FUNCTION_BLOCK FB_SENT_Decoder
VAR_INPUT
	bEnable					: BOOL;						// enable flag
	nNominalTickTimeUs		: UINT;						// nominal tick time in us
	eFastChannelConfig		: E_SentFastChnConfig;		// layout of the fast-channel data
	eSlowChannelConfig		: E_SentSlowChnConfig;		// layout of the slow-channel data
END_VAR
VAR_OUTPUT
	bNewFrameStart			: BOOL;						// indication flag new frame recieved
	nFrameLenUs				: UINT;						// frame length in µs
	
	bNewFastChnData			: BOOL;						// indication flag new new fast-channel data
	bFastChnDataValid		: BOOL;						// indication flag that the new fast-channel data are valid (CRC)
	nFastChnDataCnt			: UDINT;					// frame-counter of fast-channel data
	
	bNewSlowChnData			: BOOL;						// indication flag new new slow-channel data
	bSlowChnDataValid		: BOOL;						// indication flag that the new slow-channel data are valid (CRC)


	stRawNibbleData			: ST_SentRawNibbleData;		// raw frame data
	stFastChnData			: ST_SentFastChnData;		// last fast-channel data
	stSlowChnData			: ST_SentSlowChnData;		// last slow-channel data
	
	stRxStats				: ST_SentRxStats;			// Recieve statistic
END_VAR
VAR_IN_OUT
	nInputData				: ARRAY[*] OF BOOL;			// input data of the EL1262
END_VAR
VAR
	nMinSyncTimeUs			: UINT;						// nominal sync time - 20%
	nMaxSyncTimeUs			: UINT;						// nominal sync time + 20%
	fActTickTimeUs			: REAL;						// actual tick time (calculated from sync time)
	eFastChnCfgWork			: E_SentFastChnConfig;		// working copy of fast channel layout
	eSlowChnCfgWork			: E_SentSlowChnConfig;		// working conpy of slow channel layout
	bPausePulseWork			: BOOL;						// working copy of pause-pulse config
	nPulsesPerFrame			: UINT;						// number of pulses per send-period (including optional pause pulse)
	                                            		
	bOldValue				: BOOL;						// buffer for detection of falling edge
	bInit					: BOOL := TRUE;				// no falling edge seen yet
	                                            		
	nActSampleCnt			: UINT;						// samples since last falling edge
	nActPulseCnt			: UINT;						// pulses since last sync pulse
	                                            		
	nIdx					: DINT;						// loop-index
	                                            		
	nLowerBoundInput		: DINT;						// lowest index of input-array
	nUpperBoundInput		: DINT;						// highest index of input-array
	nCntInput				: DINT;						// number of elements in input-array
	nstate					: UINT;						// state machine variable
	
	nFastChnCrcCalc			: BYTE;						// calculated crc of fast channel data
	nSlowChnCrcCalc			: BYTE;						// calculated crc of slow channel data

	nNibbleSamples			: ARRAY[1..cMaxPulsesPerFrame] OF UINT;		// array of number of samples for each nibble
	nNibbleTicks			: ARRAY[1..cMaxPulsesPerFrame] OF USINT;	// array of number of ticks for each nibble
	
	nSlowChnBufferB2		: ARRAY[1..cMaxSlowChnLen] OF BOOL;		// Buffer for Status-Bit 2 for slow channel data
	nSlowChnBufferB3		: ARRAY[1..cMaxSlowChnLen] OF BOOL;		// Buffer for Status-Bit 3 for slow channel data
	nShortSlowChnCrcBuff	: ARRAY[1..3] OF USINT;					// Buffer to hold the short slow channel data for CRC calculation
	nEnhSlowChnCrcBuff		: ARRAY[1..4] OF USINT;					// Buffer to hold the enhanced slow channel data for CRC calculation
	
	fbTrigEnable			: Tc2_Standard.R_TRIG;		// edge detection for enable signal
	
	// Testsensor data
	
END_VAR
VAR CONSTANT
	cSyncTicks				: UINT := 56;		// number of ticks in synch pulse
	cMinFactor				: REAL := 0.8;
	cMaxFactor				: REAL := 1.2;
	cMaxPulsesPerFrame		: USINT := 10;
	cMaxSlowChnLen			: USINT := 18;
	
	// todo remove later
	cNibbleOffsetTicks		: UINT := 12;		// number of ticks in nibble für value "0"
	//cMaxNibbleTickLen		: UINT := 35;
	
END_VAR

// check edge on enable signal
fbTrigEnable(CLK:= bEnable);

IF fbTrigEnable.Q THEN
	// calculate min/max sync time
	nMinSyncTimeUs := TO_UINT(TO_REAL(nNominalTickTimeUs * cSyncTicks) * cMinFactor);
	nMaxSyncTimeUs := TO_UINT(TO_REAL(nNominalTickTimeUs * cSyncTicks) * cMaxFactor);
	
	// copy Configdata
	eFastChnCfgWork := eFastChannelConfig;	
	eSlowChnCfgWork := eSlowChannelConfig;
	
	// get number of pulses per frame
	CASE eFastChnCfgWork OF
		E_SentFastChnConfig.eValue_MsgCnt_InvMSB,
		E_SentFastChnConfig.eValue_MsgCnt_Zero,
		E_SentFastChnConfig.eValue_Value:
			nPulsesPerFrame := 9;
		
		E_SentFastChnConfig.eValueCompact:
			nPulsesPerFrame := 6;
		
		E_SentFastChnConfig.eValueExtendet:
			nPulsesPerFrame := 7;
		
	END_CASE
	
	// clear some variables
	fActTickTimeUs := 0.0;
	bInit := TRUE;
	nActPulseCnt := 0;
	Tc2_System.MEMSET(destAddr := ADR(nSlowChnBufferB2), fillByte := 0, n := SIZEOF(nSlowChnBufferB2));
	Tc2_System.MEMSET(destAddr := ADR(nSlowChnBufferB3), fillByte := 0, n := SIZEOF(nSlowChnBufferB3));
END_IF

bNewFrameStart := FALSE;
bNewFastChnData := FALSE;
bFastChnDataValid := FALSE;
bNewSlowChnData := FALSE;
bSlowChnDataValid := FALSE;


IF nInputData <> 0 THEN
	nLowerBoundInput := LOWER_BOUND(nInputData, 1);
	nUpperBoundInput := UPPER_BOUND(nInputData, 1);
	nCntInput := nUpperBoundInput - nLowerBoundInput + 1;
ELSE
	nLowerBoundInput := 0;
	nUpperBoundInput := 0;
	nCntInput := 0;
END_IF;
	
IF nCntInput > 0 THEN
	FOR nIdx := nLowerBoundInput TO nUpperBoundInput DO
		
		IF NOT bInit THEN
			nActSampleCnt := nActSampleCnt + 1;
		END_IF
		
		// check if new falling edge is detected
		IF bOldValue AND NOT nInputData[nIdx] THEN
			bInit := FALSE;
			IF nActSampleCnt > 0 THEN
				IF nMinSyncTimeUs <= nActSampleCnt AND nActSampleCnt <= nMaxSyncTimeUs THEN
					// new sync pulse detected -> clear old data					
					// calculate actual tick time from sync pulse
					fActTickTimeUs := TO_REAL(nActSampleCnt) / TO_REAL(cSyncTicks);
					bNewFrameStart := TRUE;
					nActPulseCnt := 0;
				END_IF
				
				IF fActTickTimeUs > 0.0 THEN
					nActPulseCnt := nActPulseCnt + 1;
					nNibbleSamples[nActPulseCnt] := nActSampleCnt;
					nNibbleTicks[nActPulseCnt] := TO_USINT(TO_REAL(nActSampleCnt) / fActTickTimeUs);
					
					// check if number of pulses (nibbles) is reached -> frame complet received
					IF nActPulseCnt = nPulsesPerFrame THEN
						
						// calculate frame length and update frame statistics
						nFrameLenUs := nNibbleSamples[1] + nNibbleSamples[2] + nNibbleSamples[3] + nNibbleSamples[4] + nNibbleSamples[5] + nNibbleSamples[6] + nNibbleSamples[7] + nNibbleSamples[8] + nNibbleSamples[9] + nNibbleSamples[10];
						stRxStats.nFrmRxCnt := stRxStats.nFrmRxCnt + 1;
						
						// calculate values for the nibbles and the fast channel communication
						M_CalcRawNibbleData();
						M_CalcFastChnData();
						
						bNewFastChnData := TRUE;
						bFastChnDataValid := stFastChnData.nCrc = nFastChnCrcCalc;
						
						IF bNewFastChnData AND bFastChnDataValid THEN
							stRxStats.nFrmRxCntValid := stRxStats.nFrmRxCntValid + 1;
							M_CalcSlowChnData();
						ELSIF  bNewFastChnData AND NOT bFastChnDataValid THEN
							stRxStats.nFrmRxCntInvalid := stRxStats.nFrmRxCntInvalid + 1;
							Tc2_System.MEMSET(destAddr := ADR(nSlowChnBufferB2), fillByte := 0, n := SIZEOF(nSlowChnBufferB2));
							Tc2_System.MEMSET(destAddr := ADR(nSlowChnBufferB3), fillByte := 0, n := SIZEOF(nSlowChnBufferB3));
						END_IF
					END_IF
				END_IF
				nActSampleCnt := 0;
			END_IF
		END_IF
		bOldValue := nInputData[nIdx];
	END_FOR
END_IF

METHOD PRIVATE M_CalcCrc4 : BYTE
VAR_INPUT
END_VAR
VAR_IN_OUT
	aData			: ARRAY[*] OF USINT;
END_VAR
VAR
	nLowBoundData	: DINT;			// lower index
	nUpBoundData	: DINT;			// upper index
	nIdxCntData		: DINT;			// number elements
	
	aCrc4Table 		: ARRAY[0..15] OF BYTE:=[ 0,13,7,10,14,3,9,4,1,12,6,11,15,2,8,5];		// CRC lookup table
	nIdx			: DINT;
	nRetBuff		: BYTE;
END_VAR
// check if input array is not there
IF aData <> 0 THEN
	// get array dimensions 
	nLowBoundData := LOWER_BOUND(aData, 1);
	nUpBoundData := UPPER_BOUND(aData, 1);
	IF nLowBoundData = nUpBoundData THEN
		nIdxCntData := 1;
	ELSE
		nIdxCntData := nUpBoundData - nLowBoundData + 1;	
	END_IF


	nRetBuff:=5;
	
	FOR nIdx := nLowBoundData TO nUpBoundData DO
		nRetBuff := aData[nIdx] XOR aCrc4Table[nRetBuff];
	END_FOR
	
	nRetBuff := 0 XOR aCrc4Table[nRetBuff];

END_IF

 M_CalcCrc4 := nRetBuff;
END_METHOD

METHOD PRIVATE M_CalcCrc4Legacy : BYTE
VAR_INPUT
END_VAR
VAR_IN_OUT
	aData			: ARRAY[*] OF USINT;
END_VAR
VAR
	nLowBoundData	: DINT;			// lower index
	nUpBoundData	: DINT;			// upper index
	nIdxCntData		: DINT;			// number elements
	
	aCrc4Table 		: ARRAY[0..255] OF BYTE:=[	0, 1, 2, 3, 4, 5, 6, 7, 8, 9, 10, 11, 12, 13, 14, 15,
												13, 12, 15, 14, 9, 8, 11, 10, 5, 4, 7, 6, 1, 0, 3, 2,
												7, 6, 5, 4, 3, 2, 1, 0, 15, 14, 13, 12, 11, 10, 9, 8,
												10, 11, 8, 9, 14, 15, 12, 13, 2, 3, 0, 1, 6, 7, 4, 5,
												14, 15, 12, 13, 10, 11, 8, 9, 6, 7, 4, 5, 2, 3, 0, 1,
												3, 2, 1, 0, 7, 6, 5, 4, 11, 10, 9, 8, 15, 14, 13, 12,
												9, 8, 11, 10, 13, 12, 15, 14, 1, 0, 3, 2, 5, 4, 7, 6,
												4, 5, 6, 7, 0, 1, 2, 3, 12, 13, 14, 15, 8, 9, 10, 11,
												1, 0, 3, 2, 5, 4, 7, 6, 9, 8, 11, 10, 13, 12, 15, 14,
												12, 13, 14, 15, 8, 9, 10, 11, 4, 5, 6, 7, 0, 1, 2, 3,
												6, 7, 4, 5, 2, 3, 0, 1, 14, 15, 12, 13, 10, 11, 8, 9,
												11, 10, 9, 8, 15, 14, 13, 12, 3, 2, 1, 0, 7, 6, 5, 4,
												15, 14, 13, 12, 11, 10, 9, 8, 7, 6, 5, 4, 3, 2, 1, 0,
												2, 3, 0, 1, 6, 7, 4, 5, 10, 11, 8, 9, 14, 15, 12, 13,
												8, 9, 10, 11, 12, 13, 14, 15, 0, 1, 2, 3, 4, 5, 6, 7,
												5, 4, 7, 6, 1, 0, 3, 2, 13, 12, 15, 14, 9, 8, 11, 10
												];		// CRC lookup table
	nIdx			: DINT;
	nRetBuff		: BYTE;
	temp			: BYTE;
END_VAR
// check if input array is not there
IF aData <> 0 THEN
	// get array dimensions 
	nLowBoundData := LOWER_BOUND(aData, 1);
	nUpBoundData := UPPER_BOUND(aData, 1);
	IF nLowBoundData = nUpBoundData THEN
		nIdxCntData := 1;
	ELSE
		nIdxCntData := nUpBoundData - nLowBoundData + 1;	
	END_IF


	nRetBuff:=5;
	
	FOR nIdx := nLowBoundData TO nUpBoundData DO
		temp := aData[nIdx] + (nRetBuff * 16);
		nRetBuff := aCrc4Table[temp];
	END_FOR
END_IF

 M_CalcCrc4Legacy := nRetBuff;
END_METHOD

METHOD M_CalcCrc6 : BYTE
VAR_INPUT
END_VAR
VAR_IN_OUT
	aData			: ARRAY[*] OF USINT;
END_VAR
VAR
	nLowBoundData	: DINT;			// lower index
	nUpBoundData	: DINT;			// upper index
	nIdxCntData		: DINT;			// number elements  
	
	aCrc6Table 		: ARRAY[0..63] OF BYTE:=[	0, 25, 50, 43, 61, 36, 15, 22, 35, 58, 17, 8, 30, 7, 44, 53,
												31, 6, 45, 52, 34, 59, 16, 9, 60, 37, 14, 23, 1, 24, 51, 42,
												62, 39, 12, 21, 3, 26, 49, 40, 29, 4, 47, 54, 32, 57, 18, 11,
												33, 56, 19, 10, 28, 5, 46, 55, 2, 27, 48, 41, 63, 38, 13, 20 ];		// CRC lookup table
	nIdx			: DINT;
	nRetBuff		: BYTE;
END_VAR
// check if input array is not there
IF aData <> 0 THEN
	// get array dimensions 
	nLowBoundData := LOWER_BOUND(aData, 1);
	nUpBoundData := UPPER_BOUND(aData, 1);
	IF nLowBoundData = nUpBoundData THEN
		nIdxCntData := 1;
	ELSE
		nIdxCntData := nUpBoundData - nLowBoundData + 1;	
	END_IF

	nRetBuff:=21;
	
	FOR nIdx := nLowBoundData TO nUpBoundData DO
		nRetBuff := aData[nIdx] XOR aCrc6Table[nRetBuff];
	END_FOR
	
	nRetBuff := 0 XOR aCrc6Table[nRetBuff];

END_IF

 M_CalcCrc6 := nRetBuff;
END_METHOD

METHOD PRIVATE M_CalcFastChnData
VAR_INPUT
END_VAR
CASE eFastChnCfgWork OF
	// Status (1 Nibble) + Value_1 (3 Nibble) + Messagecounter (2 Nibble) + invers MSB-Value (1 Nibble) + CRC (1 Nibble)
	E_SentFastChnConfig.eValue_MsgCnt_InvMSB:
		stFastChnData.nStatus := stRawNibbleData.nStatusValue;
		stFastChnData.nValue1 := TO_UINT(stRawNibbleData.nNibbleValue[3])
								+ ROL(TO_UINT(stRawNibbleData.nNibbleValue[2]),4)
								+ ROL(TO_UINT(stRawNibbleData.nNibbleValue[1]),8);
		stFastChnData.nMsgCnt := stRawNibbleData.nNibbleValue[5]
								+ ROL(stRawNibbleData.nNibbleValue[4],4);
		stFastChnData.nInvMsnV1 := stRawNibbleData.nNibbleValue[6];
		stFastChnData.nCrc := stRawNibbleData.nCrcValue;
		
		stFastChnData.nValue2 := 0;
		
	// Status (1 Nibble) + Value_1 (3 Nibble) + Messagecounter (2 Nibble) + Zeros (1 Nibble) + CRC (1 Nibble)
	E_SentFastChnConfig.eValue_MsgCnt_Zero:
		stFastChnData.nStatus := stRawNibbleData.nStatusValue;
		stFastChnData.nValue1 := TO_UINT(stRawNibbleData.nNibbleValue[3])
								+ ROL(TO_UINT(stRawNibbleData.nNibbleValue[2]),4)
								+ ROL(TO_UINT(stRawNibbleData.nNibbleValue[1]),8);
		stFastChnData.nMsgCnt := stRawNibbleData.nNibbleValue[5]
								+ ROL(stRawNibbleData.nNibbleValue[4],4);
		stFastChnData.nCrc := stRawNibbleData.nCrcValue;
		stFastChnData.nInvMsnV1 := 0;
		stFastChnData.nValue2 := 0;
	
	// Status (1 Nibble) + Value_1 (3 Nibble) + Value_2 (3 Nibble) + CRC (1 Nibble)
	E_SentFastChnConfig.eValue_Value:
		stFastChnData.nStatus := stRawNibbleData.nStatusValue;
		stFastChnData.nValue1 := TO_UINT(stRawNibbleData.nNibbleValue[3])
								+ ROL(TO_UINT(stRawNibbleData.nNibbleValue[2]),4)
								+ ROL(TO_UINT(stRawNibbleData.nNibbleValue[1]),8);
		stFastChnData.nValue2 := TO_UINT(stRawNibbleData.nNibbleValue[6])
								+ ROL(TO_UINT(stRawNibbleData.nNibbleValue[5]),4)
								+ ROL(TO_UINT(stRawNibbleData.nNibbleValue[4]),8);
		stFastChnData.nCrc := stRawNibbleData.nCrcValue;
		
		stFastChnData.nMsgCnt := 0;
		stFastChnData.nInvMsnV1 := 0;
	
	// Status (1 Nibble) + Value_1 (3 Nibble) + CRC (1 Nibble)	
	E_SentFastChnConfig.eValueCompact:
		stFastChnData.nStatus := stRawNibbleData.nStatusValue;
		stFastChnData.nValue1 := TO_UINT(stRawNibbleData.nNibbleValue[3])
								+ ROL(TO_UINT(stRawNibbleData.nNibbleValue[2]),4)
								+ ROL(TO_UINT(stRawNibbleData.nNibbleValue[1]),8);
		stFastChnData.nCrc := stRawNibbleData.nCrcValue;
		
		stFastChnData.nValue2 := 0;
		stFastChnData.nMsgCnt := 0;
		stFastChnData.nInvMsnV1 := 0;
		
	// Status (1 Nibble) + Value_1 (4 3bit-Nibble) + CRC (1 Nibble)
	E_SentFastChnConfig.eValueExtendet:
		stFastChnData.nStatus := stRawNibbleData.nStatusValue;
		stFastChnData.nValue1 := TO_UINT(stRawNibbleData.nNibbleValue[4])
								+ ROL(TO_UINT(stRawNibbleData.nNibbleValue[3]),3)
								+ ROL(TO_UINT(stRawNibbleData.nNibbleValue[2]),6)
								+ ROL(TO_UINT(stRawNibbleData.nNibbleValue[1]),9);
		stFastChnData.nCrc := stRawNibbleData.nCrcValue;
		
		stFastChnData.nValue2 := 0;
		stFastChnData.nMsgCnt := 0;
		stFastChnData.nInvMsnV1 := 0;
	
END_CASE

nFastChnCrcCalc := M_CalcCrc4(stRawNibbleData.nNibbleValue);
//nFastChnCrcCalc := M_CalcCrc6(stRawNibbleData.nNibbleValue);
//nFastChnCrcCalc := M_CalcCrc4Legacy(stRawNibbleData.nNibbleValue);
//nFastChnCrcCalc := M_CalcFastChnCrc_old();
END_METHOD

METHOD PRIVATE M_CalcRawNibbleData
VAR_INPUT
END_VAR
// Calculate Nibble Values
CASE eFastChnCfgWork OF
	E_SentFastChnConfig.eValue_MsgCnt_InvMSB,
	E_SentFastChnConfig.eValue_MsgCnt_Zero,
	E_SentFastChnConfig.eValue_Value:
		stRawNibbleData.nStatusTicks := nNibbleTicks[2];
		stRawNibbleData.nNibbleTicks[1] := nNibbleTicks[3];
		stRawNibbleData.nNibbleTicks[2] := nNibbleTicks[4];
		stRawNibbleData.nNibbleTicks[3] := nNibbleTicks[5];
		stRawNibbleData.nNibbleTicks[4] := nNibbleTicks[6];
		stRawNibbleData.nNibbleTicks[5] := nNibbleTicks[7];
		stRawNibbleData.nNibbleTicks[6] := nNibbleTicks[8];
		stRawNibbleData.nCrcTicks := nNibbleTicks[9];
		
		stRawNibbleData.nStatusValue := M_NibbleTicksToValue(nNibbleTicks[2]);
		stRawNibbleData.nNibbleValue[1] := M_NibbleTicksToValue(nNibbleTicks[3]);
		stRawNibbleData.nNibbleValue[2] := M_NibbleTicksToValue(nNibbleTicks[4]);
		stRawNibbleData.nNibbleValue[3] := M_NibbleTicksToValue(nNibbleTicks[5]);
		stRawNibbleData.nNibbleValue[4] := M_NibbleTicksToValue(nNibbleTicks[6]);
		stRawNibbleData.nNibbleValue[5] := M_NibbleTicksToValue(nNibbleTicks[7]);
		stRawNibbleData.nNibbleValue[6] := M_NibbleTicksToValue(nNibbleTicks[8]);
		stRawNibbleData.nCrcValue := M_NibbleTicksToValue(nNibbleTicks[9]);
		
	E_SentFastChnConfig.eValueCompact:
		stRawNibbleData.nStatusTicks := nNibbleTicks[2];
		stRawNibbleData.nNibbleTicks[1] := nNibbleTicks[3];
		stRawNibbleData.nNibbleTicks[2] := nNibbleTicks[4];
		stRawNibbleData.nNibbleTicks[3] := nNibbleTicks[5];
		stRawNibbleData.nNibbleTicks[4] := 0;
		stRawNibbleData.nNibbleTicks[5] := 0;
		stRawNibbleData.nNibbleTicks[6] := 0;
		stRawNibbleData.nCrcTicks := nNibbleTicks[6];
		
		stRawNibbleData.nStatusValue := M_NibbleTicksToValue(nNibbleTicks[2]);
		stRawNibbleData.nNibbleValue[1] := M_NibbleTicksToValue(nNibbleTicks[3]);
		stRawNibbleData.nNibbleValue[2] := M_NibbleTicksToValue(nNibbleTicks[4]);
		stRawNibbleData.nNibbleValue[3] := M_NibbleTicksToValue(nNibbleTicks[5]);
		stRawNibbleData.nNibbleValue[4] := 0;
		stRawNibbleData.nNibbleValue[5] := 0;
		stRawNibbleData.nNibbleValue[6] := 0;
		stRawNibbleData.nCrcValue := M_NibbleTicksToValue(nNibbleTicks[6]);
		
	E_SentFastChnConfig.eValueExtendet:
		stRawNibbleData.nStatusTicks := nNibbleTicks[2];
		stRawNibbleData.nNibbleTicks[1] := nNibbleTicks[3];
		stRawNibbleData.nNibbleTicks[2] := nNibbleTicks[4];
		stRawNibbleData.nNibbleTicks[3] := nNibbleTicks[5];
		stRawNibbleData.nNibbleTicks[4] := nNibbleTicks[6];
		stRawNibbleData.nNibbleTicks[5] := 0;
		stRawNibbleData.nNibbleTicks[6] := 0;
		stRawNibbleData.nCrcTicks := nNibbleTicks[7];
		
		stRawNibbleData.nStatusValue := M_NibbleTicksToValue(nNibbleTicks[2]);
		stRawNibbleData.nNibbleValue[1] := M_NibbleTicksToValue(nNibbleTicks[3]);
		stRawNibbleData.nNibbleValue[2] := M_NibbleTicksToValue(nNibbleTicks[4]);
		stRawNibbleData.nNibbleValue[3] := M_NibbleTicksToValue(nNibbleTicks[5]);
		stRawNibbleData.nNibbleValue[4] := M_NibbleTicksToValue(nNibbleTicks[6]);
		stRawNibbleData.nNibbleValue[5] := 0;
		stRawNibbleData.nNibbleValue[6] := 0;
		stRawNibbleData.nCrcValue := M_NibbleTicksToValue(nNibbleTicks[7]);
	
END_CASE
END_METHOD

METHOD PRIVATE M_CalcSlowChnData
VAR_INPUT
END_VAR
VAR
END_VAR


CASE eSlowChnCfgWork OF
	E_SentSlowChnConfig.eShortSerial:
		// shift data in buffers
		Tc2_System.MEMCPY(destAddr := ADR(nSlowChnBufferB2[1]), srcAddr := ADR(nSlowChnBufferB2[2]), n := 15);
		Tc2_System.MEMCPY(destAddr := ADR(nSlowChnBufferB3[1]), srcAddr := ADR(nSlowChnBufferB3[2]), n := 15);
		
		// insert new data
		nSlowChnBufferB2[16] := stFastChnData.nStatus.2;
		nSlowChnBufferB3[16] := stFastChnData.nStatus.3;
		
		// check if new slow channel frame is comleted
		IF nSlowChnBufferB3[1]
			AND NOT nSlowChnBufferB3[2]
			AND NOT nSlowChnBufferB3[3]
			AND NOT nSlowChnBufferB3[4]
			AND NOT nSlowChnBufferB3[5]
			AND NOT nSlowChnBufferB3[6]
			AND NOT nSlowChnBufferB3[7]
			AND NOT nSlowChnBufferB3[8]
			AND NOT nSlowChnBufferB3[9]
			AND NOT nSlowChnBufferB3[10]
			AND NOT nSlowChnBufferB3[11]
			AND NOT nSlowChnBufferB3[12]
			AND NOT nSlowChnBufferB3[13]
			AND NOT nSlowChnBufferB3[14]
			AND NOT nSlowChnBufferB3[15]
			AND NOT nSlowChnBufferB3[16] THEN
			
			bNewSlowChnData := TRUE;
			stRxStats.nSlowChnCnt := stRxStats.nSlowChnCnt + 1;
			
			// calc message id
			stSlowChnData.nMsgId := TO_USINT(nSlowChnBufferB2[4])
									+ ROL(TO_USINT(nSlowChnBufferB2[3]), 1)
									+ ROL(TO_USINT(nSlowChnBufferB2[2]), 2)
									+ ROL(TO_USINT(nSlowChnBufferB2[1]), 3);
									
			// calc data
			stSlowChnData.nData := TO_UINT(nSlowChnBufferB2[12])
									+ ROL(TO_UINT(nSlowChnBufferB2[11]), 1)
									+ ROL(TO_UINT(nSlowChnBufferB2[10]), 2)
									+ ROL(TO_UINT(nSlowChnBufferB2[9]), 3)
									+ ROL(TO_UINT(nSlowChnBufferB2[8]), 4)
									+ ROL(TO_UINT(nSlowChnBufferB2[7]), 5)
									+ ROL(TO_UINT(nSlowChnBufferB2[6]), 6)
									+ ROL(TO_UINT(nSlowChnBufferB2[5]), 7);
									
			// calc crc
			stSlowChnData.nCrc := TO_USINT(nSlowChnBufferB2[16])
									+ ROL(TO_USINT(nSlowChnBufferB2[15]), 1)
									+ ROL(TO_USINT(nSlowChnBufferB2[14]), 2)
									+ ROL(TO_USINT(nSlowChnBufferB2[13]), 3);
									
			// CRC-Check
			// clear buffer
			Tc2_System.MEMSET(destAddr := ADR(nShortSlowChnCrcBuff), fillByte := 0, n := SIZEOF(nShortSlowChnCrcBuff));
			
			// build buffer
			nShortSlowChnCrcBuff[1].0 := nSlowChnBufferB2[4];
			nShortSlowChnCrcBuff[1].1 := nSlowChnBufferB2[3];
			nShortSlowChnCrcBuff[1].2 := nSlowChnBufferB2[2];
			nShortSlowChnCrcBuff[1].3 := nSlowChnBufferB2[1];
			
			nShortSlowChnCrcBuff[2].0 := nSlowChnBufferB2[8];
			nShortSlowChnCrcBuff[2].1 := nSlowChnBufferB2[7];
			nShortSlowChnCrcBuff[2].2 := nSlowChnBufferB2[6];
			nShortSlowChnCrcBuff[2].3 := nSlowChnBufferB2[5];
			
			nShortSlowChnCrcBuff[3].0 := nSlowChnBufferB2[12];
			nShortSlowChnCrcBuff[3].1 := nSlowChnBufferB2[11];
			nShortSlowChnCrcBuff[3].2 := nSlowChnBufferB2[10];
			nShortSlowChnCrcBuff[3].3 := nSlowChnBufferB2[9];
			
			// calc crc value of transmitted data
			nSlowChnCrcCalc := M_CalcCrc4(nShortSlowChnCrcBuff);
			
			bSlowChnDataValid := nSlowChnCrcCalc = stSlowChnData.nCrc;

			IF bSlowChnDataValid THEN
				stRxStats.nSlowChnCntValid := stRxStats.nSlowChnCntValid + 1;
			ELSE
				stRxStats.nSlowChnCntInvalid := stRxStats.nSlowChnCntInvalid + 1;
			END_IF
		
		END_IF
		
	E_SentSlowChnConfig.eEnhancedSerial:
		// shift data in buffers
		Tc2_System.MEMCPY(destAddr := ADR(nSlowChnBufferB2[1]), srcAddr := ADR(nSlowChnBufferB2[2]), n := 17);
		Tc2_System.MEMCPY(destAddr := ADR(nSlowChnBufferB3[1]), srcAddr := ADR(nSlowChnBufferB3[2]), n := 17);
		
		// insert new data
		nSlowChnBufferB2[18] := stFastChnData.nStatus.2;
		nSlowChnBufferB3[18] := stFastChnData.nStatus.3;
		
		// check if new slow channel frame is comleted
		IF nSlowChnBufferB3[1]
			AND nSlowChnBufferB3[2]
			AND nSlowChnBufferB3[3]
			AND nSlowChnBufferB3[4]
			AND nSlowChnBufferB3[5]
			AND nSlowChnBufferB3[6]
			AND NOT nSlowChnBufferB3[7]
			AND NOT nSlowChnBufferB3[13]
			AND NOT nSlowChnBufferB3[18] THEN
			
			
			bNewSlowChnData := TRUE;
			stRxStats.nSlowChnCnt := stRxStats.nSlowChnCnt + 1;
			
			// check which enhanced serial format is used
			IF NOT nSlowChnBufferB3[8] THEN
				// 12-bit data format
				
				// calc message id
				stSlowChnData.nMsgId := TO_USINT(nSlowChnBufferB3[17])
										+ ROL(TO_USINT(nSlowChnBufferB3[16]), 1)
										+ ROL(TO_USINT(nSlowChnBufferB3[15]), 2)
										+ ROL(TO_USINT(nSlowChnBufferB3[14]), 3)
										+ ROL(TO_USINT(nSlowChnBufferB3[12]), 4)
										+ ROL(TO_USINT(nSlowChnBufferB3[11]), 5)
										+ ROL(TO_USINT(nSlowChnBufferB3[10]), 6)
										+ ROL(TO_USINT(nSlowChnBufferB3[9]), 7);
				
				// calc data
				stSlowChnData.nData := TO_UINT(nSlowChnBufferB2[18])
										+ ROL(TO_UINT(nSlowChnBufferB2[17]), 1)
										+ ROL(TO_UINT(nSlowChnBufferB2[16]), 2)
										+ ROL(TO_UINT(nSlowChnBufferB2[15]), 3)
										+ ROL(TO_UINT(nSlowChnBufferB2[14]), 4)
										+ ROL(TO_UINT(nSlowChnBufferB2[13]), 5)
										+ ROL(TO_UINT(nSlowChnBufferB2[12]), 6)
										+ ROL(TO_UINT(nSlowChnBufferB2[11]), 7)
										+ ROL(TO_UINT(nSlowChnBufferB2[10]), 8)
										+ ROL(TO_UINT(nSlowChnBufferB2[9]), 9)
										+ ROL(TO_UINT(nSlowChnBufferB2[8]), 10)
										+ ROL(TO_UINT(nSlowChnBufferB2[7]), 11);
										
			ELSE
				// 16-bit data format
				// calc message id
				stSlowChnData.nMsgId := TO_USINT(nSlowChnBufferB3[12])
										+ ROL(TO_USINT(nSlowChnBufferB3[11]), 1)
										+ ROL(TO_USINT(nSlowChnBufferB3[10]), 2)
										+ ROL(TO_USINT(nSlowChnBufferB3[9]), 3);
				
				// calc data
				stSlowChnData.nData := TO_UINT(nSlowChnBufferB2[18])
										+ ROL(TO_UINT(nSlowChnBufferB2[17]), 1)
										+ ROL(TO_UINT(nSlowChnBufferB2[16]), 2)
										+ ROL(TO_UINT(nSlowChnBufferB2[15]), 3)
										+ ROL(TO_UINT(nSlowChnBufferB2[14]), 4)
										+ ROL(TO_UINT(nSlowChnBufferB2[13]), 5)
										+ ROL(TO_UINT(nSlowChnBufferB2[12]), 6)
										+ ROL(TO_UINT(nSlowChnBufferB2[11]), 7)
										+ ROL(TO_UINT(nSlowChnBufferB2[10]), 8)
										+ ROL(TO_UINT(nSlowChnBufferB2[9]), 9)
										+ ROL(TO_UINT(nSlowChnBufferB2[8]), 10)
										+ ROL(TO_UINT(nSlowChnBufferB2[7]), 11)
										+ ROL(TO_UINT(nSlowChnBufferB3[17]), 12)
										+ ROL(TO_UINT(nSlowChnBufferB3[16]), 13)
										+ ROL(TO_UINT(nSlowChnBufferB3[15]), 14)
										+ ROL(TO_UINT(nSlowChnBufferB3[14]), 15);
			END_IF
			
				
									
			// calc crc
			stSlowChnData.nCrc := TO_USINT(nSlowChnBufferB2[6])
									+ ROL(TO_USINT(nSlowChnBufferB2[5]), 1)
									+ ROL(TO_USINT(nSlowChnBufferB2[4]), 2)
									+ ROL(TO_USINT(nSlowChnBufferB2[3]), 3)
									+ ROL(TO_USINT(nSlowChnBufferB2[2]), 4)
									+ ROL(TO_USINT(nSlowChnBufferB2[1]), 5);
									
			// CRC-Check
			// clear buffer
			Tc2_System.MEMSET(destAddr := ADR(nEnhSlowChnCrcBuff), fillByte := 0, n := SIZEOF(nEnhSlowChnCrcBuff));
			
			// build buffer
			nEnhSlowChnCrcBuff[1].5 := nSlowChnBufferB2[7];
			nEnhSlowChnCrcBuff[1].4 := nSlowChnBufferB3[7];
			nEnhSlowChnCrcBuff[1].3 := nSlowChnBufferB2[8];
			nEnhSlowChnCrcBuff[1].2 := nSlowChnBufferB3[8];
			nEnhSlowChnCrcBuff[1].1 := nSlowChnBufferB2[9];
			nEnhSlowChnCrcBuff[1].0 := nSlowChnBufferB3[9];
			
			nEnhSlowChnCrcBuff[2].5 := nSlowChnBufferB2[10];
			nEnhSlowChnCrcBuff[2].4 := nSlowChnBufferB3[10];
			nEnhSlowChnCrcBuff[2].3 := nSlowChnBufferB2[11];
			nEnhSlowChnCrcBuff[2].2 := nSlowChnBufferB3[11];
			nEnhSlowChnCrcBuff[2].1 := nSlowChnBufferB2[12];
			nEnhSlowChnCrcBuff[2].0 := nSlowChnBufferB3[12];
			
			nEnhSlowChnCrcBuff[3].5 := nSlowChnBufferB2[13];
			nEnhSlowChnCrcBuff[3].4 := nSlowChnBufferB3[13];
			nEnhSlowChnCrcBuff[3].3 := nSlowChnBufferB2[14];
			nEnhSlowChnCrcBuff[3].2 := nSlowChnBufferB3[14];
			nEnhSlowChnCrcBuff[3].1 := nSlowChnBufferB2[15];
			nEnhSlowChnCrcBuff[3].0 := nSlowChnBufferB3[15];
			
			nEnhSlowChnCrcBuff[4].5 := nSlowChnBufferB2[16];
			nEnhSlowChnCrcBuff[4].4 := nSlowChnBufferB3[16];
			nEnhSlowChnCrcBuff[4].3 := nSlowChnBufferB2[17];
			nEnhSlowChnCrcBuff[4].2 := nSlowChnBufferB3[17];
			nEnhSlowChnCrcBuff[4].1 := nSlowChnBufferB2[18];
			nEnhSlowChnCrcBuff[4].0 := nSlowChnBufferB3[18];
			
			// calc crc value of transmitted data
			nSlowChnCrcCalc := M_CalcCrc6(nEnhSlowChnCrcBuff);
			
			bSlowChnDataValid := nSlowChnCrcCalc = stSlowChnData.nCrc;
			
			IF bSlowChnDataValid THEN
				stRxStats.nSlowChnCntValid := stRxStats.nSlowChnCntValid + 1;
			ELSE
				stRxStats.nSlowChnCntInvalid := stRxStats.nSlowChnCntInvalid + 1;
			END_IF
				
		END_IF
END_CASE
END_METHOD

METHOD PRIVATE M_NibbleTicksToValue : USINT
VAR_INPUT
	nNibbleTicks		: USINT;
END_VAR
VAR
	nValue				: USINT;
END_VAR
CASE nNibbleTicks OF
	0..12: nValue:=0;
	13:nValue:=1;
	14:nValue:=2;
	15:nValue:=3;
	16:nValue:=4;
	17:nValue:=5;
	18:nValue:=6;
	19:nValue:=7;
	20:nValue:=8;
	21:nValue:=9;
	22:nValue:=16#A;
	23:nValue:=16#B;
	24:nValue:=16#C;
	25:nValue:=16#D;
	26:nValue:=16#E;
	27..28:nValue:=16#F;
END_CASE

M_NibbleTicksToValue := nValue;
END_METHOD

METHOD M_ResetStats
VAR_INPUT
END_VAR
stRxStats.nFrmRxCnt := 0;
stRxStats.nFrmRxCntInvalid := 0;
stRxStats.nFrmRxCntValid := 0;
stRxStats.nSlowChnCnt := 0;
stRxStats.nSlowChnCntInvalid := 0;
stRxStats.nSlowChnCntValid := 0;
END_METHOD

END_FUNCTION_BLOCK
